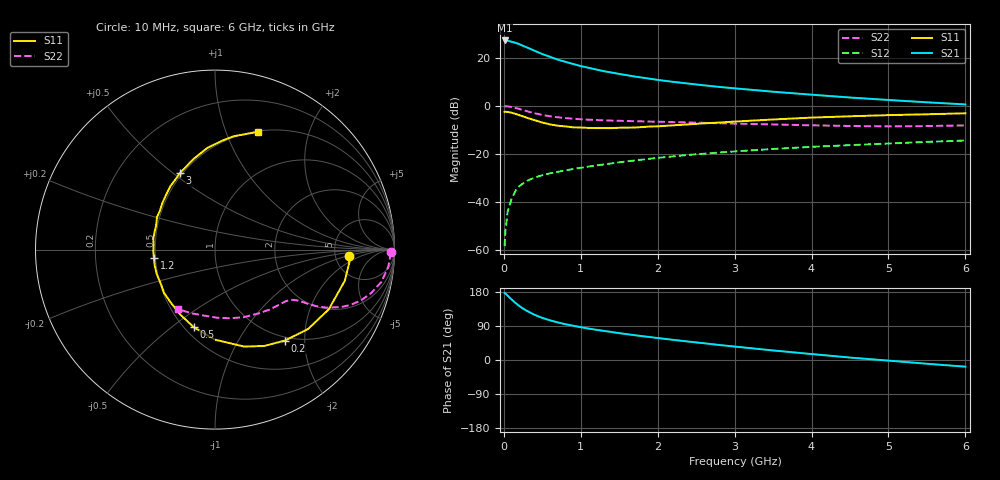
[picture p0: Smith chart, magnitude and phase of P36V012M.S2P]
! SIEMENS Small Signal Semiconductors
! BFP181
! Si NPN RF Bipolar Junction Transistor in SOT143
! VCE = 6 V  IC = 12 mA
! Common Emitter S-Parameters:  March  1996
# GHz  S  MA  R  50
!  f  S11  S21  S12  S22
! GHz  MAG  ANG  MAG  ANG  MAG  ANG  MAG  ANG
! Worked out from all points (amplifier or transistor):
!   36 points, 10 MHz to 6 GHz, reference 50 ohm
!   highest |S21| = 27.2 dB at 10 MHz (marker M1)
!   |S21| within 3 dB of that: start of sweep to 307.9 MHz
!   unconditionally stable (mu >= 1): 1.172 GHz to end of sweep
!   at 250 MHz: K = 0.35, MSG = 28.6 dB, |S12| = -32.3 dB
!   at 1.4 GHz: K = 1.07, MAG = 17.3 dB, |S12| = -24.0 dB
!   at 6 GHz: K = 1.01, MAG = 6.8 dB, |S12| = -14.4 dB
!   S11 on the Smith chart (normalised r, x): 10 MHz: 6.76, -1.17; 200 MHz: 0.94, -1.61; 500 MHz: 0.56, -0.60; 1.2 GHz: 0.49, -0.05; 3 GHz: 0.48, +0.53; 6 GHz: 0.51, +1.30
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0.01  0.7488 -2.9  22.89 177.1  0.0012 85.5  0.9785 -0.9
0.02  0.7517 -5.6  22.83 175.7  0.0024 85.5  0.9773 -2.1
0.05  0.7437 -13.5  22.55 169.7  0.0064 85.7  0.9705 -5.6
0.1  0.716 -27.7  21.54 160.0  0.0115 75.9  0.9452 -10.9
0.15  0.6816 -40.5  20.48 150.8  0.0169 70.3  0.9036 -15.5
0.2  0.6395 -52.4  19.2 142.8  0.0212 66.5  0.8599 -19.3
0.25  0.6028 -63.0  17.69 135.5  0.0243 62.5  0.814 -22.3
0.3  0.564 -73.3  16.41 129.7  0.0274 59.3  0.7717 -24.5
0.4  0.5015 -90.2  13.96 119.2  0.0321 55.6  0.7007 -27.5
0.5  0.4481 -105.4  11.93 111.1  0.0359 52.5  0.6457 -29.2
0.6  0.4109 -117.9  10.46 104.7  0.0394 51.8  0.606 -30.1
0.7  0.3852 -129.5  9.141 99.2  0.0422 51.4  0.5767 -30.7
0.9  0.3565 -148.2  7.425 90.5  0.0484 50.5  0.5382 -31.7
1.1  0.3473 -165.2  6.182 82.9  0.0543 50.4  0.5138 -33.0
1.2  0.3436 -172.0  5.684 79.8  0.0574 50.4  0.5061 -33.8
1.7  0.3536 158.7  4.073 65.5  0.0727 49.7  0.4782 -38.6
2.2  0.392 138.3  3.154 53.2  0.0885 47.2  0.4578 -45.0
3  0.4696 114.4  2.31 35.5  0.1124 41.8  0.4255 -57.5
3.5  0.519 103.3  1.964 25.2  0.1264 38.3  0.4093 -66.8
4.5  0.605 86.8  1.487 6.4  0.1519 30.2  0.38 -88.1
5.5  0.666 75.1  1.182 -9.9  0.1776 23.0  0.379 -110.7
6  0.698 70.0  1.068 -17.6  0.1895 19.0  0.3904 -122.2
